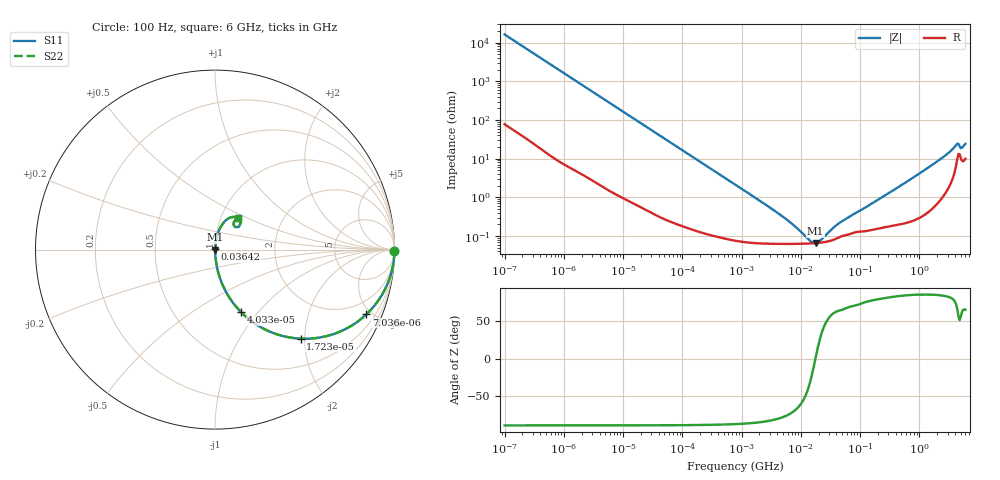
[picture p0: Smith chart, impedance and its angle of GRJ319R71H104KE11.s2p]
!Murata Part Number: GRJ319R71H104KE11
!These Parameters are Measured in Series Mode Connection
!Data Generated on Jun 19, 2026
!  o--ll--o
!Port1  Port2
!  o------o
!Operation Temp=25[degC], DC Bias Voltage=0[V]
!Freq. Start=100[Hz] Stop=6[GHz] 401[Steps]
# Hz S RI R 50
!Freq.(Hz) S11(Real) S11(Imag) S21(Real) S21(Imag) S12(Real) S12(Imag) S22(Real) S22(Imag)
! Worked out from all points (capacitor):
!   401 points, 100 Hz to 6 GHz, reference 50 ohm
!   read as one part in series: C = 98.2 nF near 109 Hz
!   lowest |Z| = 65.8 mohm at 17.79 MHz (marker M1)
!   series resonance near 17.64 MHz, so ESL is about 830 pH
!   S11 on the Smith chart (normalised r, x): 100 Hz: open; 7.036 kHz: 1.03, -4.66; 17.23 kHz: 1.01, -1.91; 40.34 kHz: 1.01, -0.82; 36.42 MHz: 1.00, +0.00; 6 GHz: 1.20, +0.44
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100  0.9999 -0.00618  6.79e-05 0.00618  6.79e-05 0.00618  0.9999 -0.00618
627  0.9984 -0.0385  0.00165 0.0385  0.00165 0.0385  0.9984 -0.0385
2008  0.9845 -0.1211  0.0155 0.1211  0.0155 0.1211  0.9845 -0.1211
4111  0.9395 -0.2358  0.0605 0.2358  0.0605 0.2358  0.9395 -0.2358
7036  0.8429 -0.3611  0.1571 0.3611  0.1571 0.3611  0.8429 -0.3611
11514  0.6692 -0.4675  0.3308 0.4675  0.3308 0.4675  0.6692 -0.4675
17227  0.4766 -0.4962  0.5234 0.4962  0.5234 0.4962  0.4766 -0.4962
26957  0.2731 -0.442  0.7269 0.442  0.7269 0.442  0.2731 -0.442
40335  0.1451 -0.3484  0.8549 0.3484  0.8549 0.3484  0.1451 -0.3484
69028  0.056 -0.2254  0.944 0.2254  0.944 0.2254  0.056 -0.2254
141303  0.015 -0.1154  0.985 0.1154  0.985 0.1154  0.015 -0.1154
774597  0.00122 -0.0215  0.9988 0.0215  0.9988 0.0215  0.00122 -0.0215
5311619  0.000635 -0.00287  0.9994 0.00287  0.9994 0.00287  0.000635 -0.00287
1.555665e7  0.000649 -0.00024  0.9994 0.00024  0.9994 0.00024  0.000649 -0.00024
1.779312e7  0.000657 1.62e-05  0.9993 -1.62e-05  0.9993 -1.62e-05  0.000657 1.62e-05
2.128304e7  0.000675 0.000359  0.9993 -0.000359  0.9993 -0.000359  0.000675 0.000359
3.64232e7  0.000814 0.00149  0.9992 -0.00149  0.9992 -0.00149  0.000814 0.00149
3.124326e8  0.00194 0.013  0.9981 -0.013  0.9981 -0.013  0.00194 0.013
2.34314e9  0.0186 0.0975  0.9814 -0.0975  0.9814 -0.0975  0.0186 0.0975
4.193612e9  0.1004 0.1822  0.8996 -0.1822  0.8996 -0.1822  0.1004 0.1822
5.245841e9  0.103 0.1398  0.897 -0.1398  0.897 -0.1398  0.103 0.1398
6e9  0.1259 0.175  0.8741 -0.175  0.8741 -0.175  0.1259 0.175
